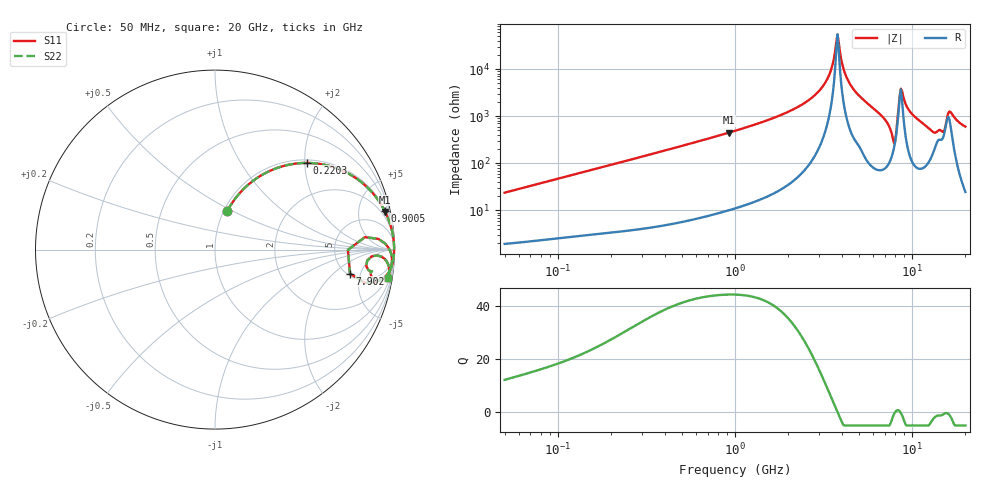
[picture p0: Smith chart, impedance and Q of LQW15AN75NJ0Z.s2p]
!Murata Part Number: LQW15AN75NJ0Z
!These Parameters are Measured in Series Mode Connection
!  o--[Z]--o
!Port1  Port2
!  o-------o
!Freq. Start=50[MHz] Stop=20[GHz], 401[Steps]
# Hz S RI R 50
!Freq.(Hz) S11(Real) S11(Imag) S21(Real) S21(Imag) S12(Real) S12(Imag) S22(Real) S22(Imag)
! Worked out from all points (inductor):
!   401 points, 50 MHz to 20 GHz, reference 50 ohm
!   read as one part in series: L = 75.2 nH near 51.52 MHz
!   highest Q = 44.3 at 927.8 MHz (marker M1), where L = 77 nH
!   self-resonance near 3.736 GHz
!   S11 on the Smith chart (normalised r, x): 50 MHz: 1.04, +0.47; 220.3 MHz: 1.07, +2.04; 900.5 MHz: 1.20, +8.69; 7.902 GHz: 5.25, -3.37; 20 GHz: 1, -12
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5e7  0.0695 0.2166  0.9305 -0.2166  0.9305 -0.2166  0.0695 0.2166
1.364002e8  0.297 0.4346  0.703 -0.4346  0.703 -0.4346  0.297 0.4346
2.202824e8  0.5109 0.4829  0.4891 -0.4829  0.4891 -0.4829  0.5109 0.4829
3.721004e8  0.7437 0.4235  0.2563 -0.4235  0.2563 -0.4235  0.7437 0.4235
9.00459e8  0.9453 0.2163  0.0547 -0.2163  0.0547 -0.2163  0.9453 0.2163
9.278425e8  0.9485 0.21  0.0515 -0.21  0.0515 -0.21  0.9485 0.21
1e9  0.9558 0.1946  0.0442 -0.1946  0.0442 -0.1946  0.9558 0.1946
2.728004e9  0.9965 0.0398  0.00346 -0.0398  0.00346 -0.0398  0.9965 0.0398
3.364474e9  0.998 0.0145  0.002 -0.0145  0.002 -0.0145  0.998 0.0145
3.792786e9  0.9982 -1.22e-05  0.00185 1.22e-05  0.00185 1.22e-05  0.9982 -1.22e-05
4.149438e9  0.9979 -0.0112  0.00211 0.0112  0.00211 0.0112  0.9979 -0.0112
4.539627e9  0.9972 -0.0229  0.00285 0.0229  0.00285 0.0229  0.9972 -0.0229
7.442007e9  0.9468 -0.1525  0.0532 0.1525  0.0532 0.1525  0.9468 -0.1525
7.901521e9  0.7522 -0.1338  0.2478 0.1338  0.2478 0.1338  0.7522 -0.1338
8.141811e9  0.8349 0.0693  0.1651 -0.0693  0.1651 -0.0693  0.8349 0.0693
8.516016e9  0.9659 0.0113  0.0341 -0.0113  0.0341 -0.0113  0.9659 0.0113
8.774992e9  0.9807 -0.0215  0.0193 0.0215  0.0193 0.0215  0.9807 -0.0215
9.892087e9  0.9842 -0.0837  0.0158 0.0837  0.0158 0.0837  0.9842 -0.0837
1.295331e10  0.9095 -0.1699  0.0905 0.1699  0.0905 0.1699  0.9095 -0.1699
1.482269e10  0.8554 -0.1144  0.1446 0.1144  0.1446 0.1144  0.8554 -0.1144
1.646126e10  0.9548 -0.0632  0.0452 0.0632  0.0452 0.0632  0.9548 -0.0632
2e10  0.9666 -0.1604  0.0334 0.1604  0.0334 0.1604  0.9666 -0.1604
